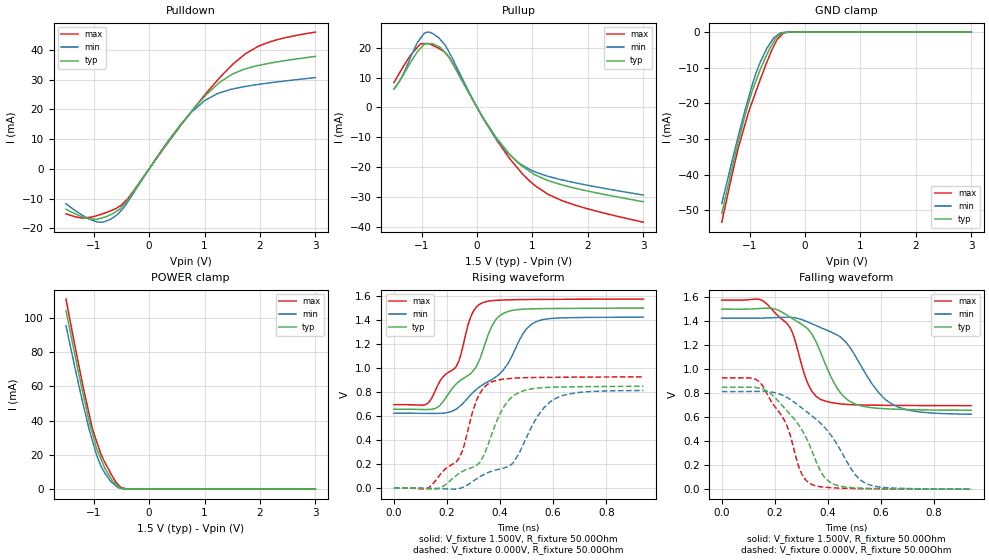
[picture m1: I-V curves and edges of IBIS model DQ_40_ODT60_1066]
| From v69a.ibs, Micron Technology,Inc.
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| MODEL DQ_40_ODT60_1066 (40 Ohm Data I/O with 60ohm ODT, 800/1066Mbps)
[Model]   DQ_40_ODT60_1066
Model_type   I/O
Vinl = 575.000mV
Vinh = 925.000mV
Vmeas = 750.000mV
Vref = 750.000mV
Cref = 0.0pF
Rref = 25.000Ohm
|   typ   min   max
C_comp   1.26pF   1.11pF   1.44pF
| Note: C_comp changes when the ODT circuit is enabled.
[Model Spec]
| Input threshold voltage corners
Vinl   0.5750V   0.5375V   0.6125V
Vinh   0.9250V   0.8875V   0.9625V
| Measurement voltage corners
Vmeas   0.7500V   0.7125V   0.7875V
| Timing spec test load voltage corners
Vref   0.7500V   0.7125V   0.7875V
[Receiver Thresholds]
Vth   =  0.750V
Vth_min  =  0.735V
Vth_max  =  0.765V
Vinh_ac  =  0.175V
Vinh_dc  =  0.100V
Vinl_ac  = -0.175V
Vinl_dc  = -0.100V
Tslew_ac =  5.000ns |Not specified, so set to high value
Threshold_sensitivity = 0.50
Reference_supply Pullup_ref
[Voltage Range]   1.5000V   1.4250V   1.5750V
[Pullup Reference]   1.5000V   1.4250V   1.5750V
| Junction Temperature (Ambient temp is 35C typ, 95C min, 0C max)
[Temperature Range]   50.0   110.0   0.0
[Add Submodel]
| Submodel Name   Mode
60ohm_ODT_1066   Non-Driving
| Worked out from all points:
|   slope of the pulldown table from 0 to 0.225 V, typ, clamps not added: 37.3 ohm
|   slope of the pullup table from 0 to 0.225 V, typ, clamps not added: 33.3 ohm
|   GND clamp passes 1 mA (typ) near -0.48 V on its own axis
|   POWER clamp passes 1 mA (typ) near -0.54 V on its own axis
|   falling waveform, V_fixture 1.500V, R_fixture 50.00Ohm: 20-80 % time 114ps typ, 151ps min, 90.5ps max; typ from 1.5 V to 0.657 V
|   rising waveform, V_fixture 1.500V, R_fixture 50.00Ohm: 20-80 % time 147ps typ, 188ps min, 116ps max; typ from 0.657 V to 1.5 V
|   rising waveform, V_fixture 0.000V, R_fixture 50.00Ohm: 20-80 % time 123ps typ, 153ps min, 104ps max; typ from 0 V to 0.848 V
|   falling waveform, V_fixture 0.000V, R_fixture 50.00Ohm: 20-80 % time 133ps typ, 173ps min, 107ps max; typ from 0.848 V to 0 V
[Pulldown]
|   Voltage   I(typ)   I(min)   I(max)
-1.5V     -13.6mA    -11.75mA   -15.12mA
-1.195V   -16.21mA   -15.72mA   -16.58mA
-960mV    -16.98mA   -17.75mA   -15.83mA
-690mV    -15.38mA   -16.91mA   -14.11mA
-530mV    -13.56mA   -14.54mA   -12.57mA
-380mV    -10.33mA   -10.94mA   -9.938mA
540mV     14.03mA    14.24mA    13.81mA
1V        24.29mA    22.9mA     24.74mA
1.265V    28.96mA    25.48mA    30.46mA
1.495V    31.78mA    26.77mA    34.87mA
1.97V     34.74mA    28.36mA    41.2mA
3V        37.78mA    30.67mA    45.95mA
[GND Clamp]
|   Voltage   I(typ)   I(min)   I(max)
-1.5V     -50.86mA   -48.03mA   -53.31mA
-1.32V    -38.49mA   -36.47mA   -40.31mA
-1.195V   -30.28mA   -28.67mA   -32mA
-1.085V   -23.47mA   -22.1mA    -26.06mA
-950mV    -16.36mA   -14.72mA   -19.5mA
-875mV    -13.3mA    -11.18mA   -16.21mA
-805mV    -10.44mA   -8.35mA    -13.23mA
-690mV    -6.381mA   -4.61mA    -8.515mA
-565mV    -2.71mA    -1.629mA   -4.002mA
-505mV    -1.389mA   -935.1uA   -2.13mA
-380mV    -171.4uA   -110.2uA   -180.2uA
3V        0A         0A         0A
[Pullup]
|   Voltage   I(typ)   I(min)   I(max)
-1.5V     6.153mA    6.385mA    8.388mA
-1.365V   9.878mA    9.978mA    12.67mA
-1.025V   19.77mA    23.13mA    21.32mA
-835mV    21.43mA    25.16mA    21.21mA
-660mV    20.15mA    22.79mA    19.54mA
-505mV    16.8mA     18.6mA     16.93mA
80mV      -2.482mA   -2.723mA   -2.581mA
310mV     -9.086mA   -9.637mA   -9.633mA
770mV     -19.05mA   -18.9mA    -21.22mA
1.055V    -22.71mA   -21.69mA   -26.38mA
1.51V     -25.9mA    -24.24mA   -31.14mA
3V        -31.67mA   -29.44mA   -38.55mA
[POWER Clamp]
|   Voltage   I(typ)   I(min)   I(max)
-1.5V     104.2mA    95.33mA    110.8mA
-1.195V   56.08mA    50.05mA    60.2mA
-1.09V    40.77mA    35.95mA    44.95mA
-1.025V   32.84mA    28.43mA    35.51mA
-950mV    23.76mA    20.16mA    28.1mA
-870mV    17.62mA    13.67mA    20.38mA
-795mV    11.95mA    9.2mA      15.38mA
-690mV    6.402mA    4.437mA    8.988mA
-595mV    2.805mA    1.754mA    3.913mA
-505mV    588.2uA    491.1uA    931.8uA
-300mV    1.53uA     2.94uA     1.674uA
3V        0A         0A         0A
[Ramp]
R_load = 50.00Ohm
|   typ   min   max
dV/dt_r   508.798mV/123.002ps 487.677mV/153.142ps 555.841mV/104.138ps
dV/dt_f   504.967mV/113.836ps 479.854mV/151.141ps 527.439mV/90.495ps
[Falling Waveform]
V_fixture = 1.500V
V_fixture_min = 1.425V
V_fixture_max = 1.575V
R_fixture = 50.00Ohm
|   Time   V(typ)   V(min)   V(max)
0s        1.499V     1.424V     1.574V
145ps     1.505V     1.424V     1.578V
245ps     1.45V      1.431V     1.381V
270ps     1.415V     1.428V     1.279V
325ps     1.332V     1.392V     875.9mV
370ps     1.151V     1.348V     749.8mV
435ps     838.6mV    1.283V     714.1mV
500ps     711.1mV    1.12V      703mV
640ps     667.3mV    710.7mV    697.8mV
940ps     657.2mV    623.8mV    695.1mV
[Rising Waveform]
V_fixture = 1.500V
V_fixture_min = 1.425V
V_fixture_max = 1.575V
R_fixture = 50.00Ohm
|   Time   V(typ)   V(min)   V(max)
0s        657.2mV    623.8mV    695.1mV
130ps     655.3mV    622.6mV    710.5mV
185ps     719.7mV    624.8mV    926.5mV
235ps     868.8mV    658.2mV    1.014V
290ps     955.1mV    778.4mV    1.428V
335ps     1.147V     861.3mV    1.544V
400ps     1.437V     956.1mV    1.565V
485ps     1.489V     1.281V     1.57V
540ps     1.494V     1.39V      1.571V
940ps     1.499V     1.424V     1.574V
[Rising Waveform]
V_fixture = 0.000V
V_fixture_min = 0.000V
V_fixture_max = 0.000V
R_fixture = 50.00Ohm
|   Time   V(typ)   V(min)   V(max)
0s        250uV      307.8uV    134.6uV
130ps     -5.431mV   -289.2uV   2.591mV
235ps     105.8mV    -7.022mV   219.4mV
260ps     142.1mV    7.733mV    323.5mV
310ps     187.3mV    75.89mV    725.3mV
370ps     457.2mV    142.1mV    886.4mV
455ps     776.4mV    230.8mV    916.6mV
540ps     832.8mV    594.1mV    921.6mV
615ps     841.6mV    754.1mV    923.1mV
940ps     848.2mV    813.1mV    926.5mV
[Falling Waveform]
V_fixture = 0.000V
V_fixture_min = 0.000V
V_fixture_max = 0.000V
R_fixture = 50.00Ohm
|   Time   V(typ)   V(min)   V(max)
0s        848.2mV    813.1mV    926.5mV
145ps     839.2mV    814.2mV    885mV
235ps     677.9mV    776.4mV    576.3mV
275ps     578.1mV    720.9mV    302.7mV
300ps     498.6mV    678.4mV    132.5mV
340ps     316.7mV    609.5mV    38.8mV
410ps     55.34mV    453.9mV    12.38mV
500ps     11.17mV    128.3mV    5.346mV
540ps     7.65mV     51.18mV    4.149mV
940ps     250uV      307.8uV    134.6uV
